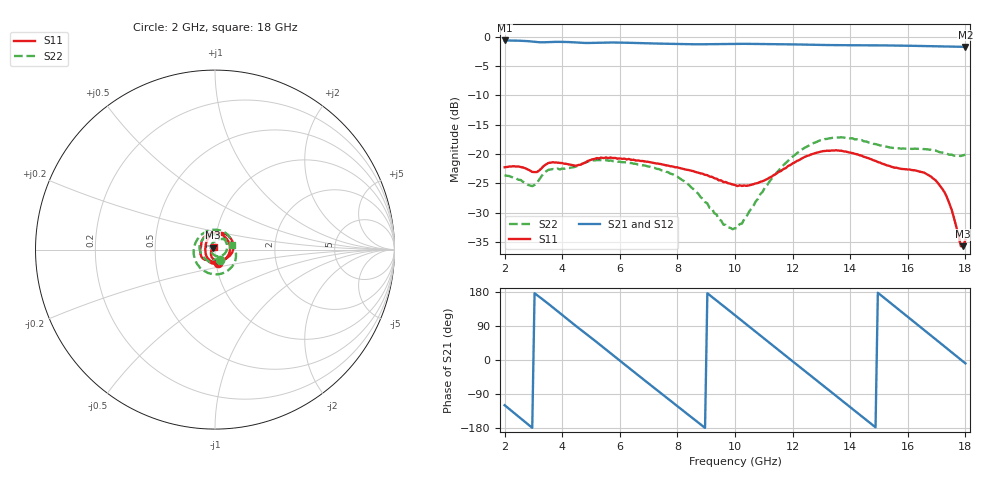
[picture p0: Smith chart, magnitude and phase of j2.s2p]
!Keysight Technologies,P5004A,MY58100454,A.15.10.06
!Date: Monday, July 18, 2022 10:32:16
!Correction: S11(C  2-Port  )
!S21(C  2-Port  )
!S12(C  2-Port  )
!S22(C  2-Port  )
!S2P File: Measurements: S11, S21, S12, S22:
# Hz S  dB  R 50
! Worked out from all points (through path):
!   201 points, 2 GHz to 18 GHz, reference 50 ohm
!   highest |S21| = -0.66 dB at 2 GHz (marker M1); lowest = -1.8 dB at 18 GHz (marker M2)
!   group delay of S21, straight-line fit = 168 ps
!   lowest |S11| = -35.7 dB at 17.92 GHz (marker M3), VSWR 1.03, Z = 48.7 + j1.01 ohm
!   |S11| at or under -10 dB: start of sweep to end of sweep
!   |S22| runs from -32.8 to -17.2 dB; largest |S21 - S12| = 0.00052
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2e9  -22.24 -76.1  -0.66 -119.2  -0.66 -119.2  -23.60 -63.9
2.64e9  -22.28 -111.1  -0.73 -159.1  -0.73 -159.1  -24.73 -89.6
3.2e9  -22.79 -128.3  -0.96 166.9  -0.96 166.9  -24.35 -94.0
4e9  -21.54 -171.1  -0.90 118.9  -0.90 118.9  -22.45 -137.3
4.72e9  -21.59 157.1  -1.08 75.3  -1.08 75.3  -21.58 -173.3
6e9  -20.73 79.7  -1.02 -1.5  -1.02 -1.6  -21.29 109.0
6.56e9  -21.11 45.0  -1.09 -35.6  -1.09 -35.6  -21.66 77.0
7.36e9  -21.64 -5.7  -1.19 -83.6  -1.19 -83.6  -22.56 31.8
8e9  -22.27 -47.1  -1.26 -122.0  -1.26 -122.0  -23.85 -6.1
8.8e9  -23.29 -100.2  -1.31 -169.6  -1.31 -169.6  -27.28 -57.8
1e10  -25.25 -169.0  -1.24 118.2  -1.24 118.2  -32.62 -173.7
1.072e10  -25.00 160.4  -1.25 74.4  -1.25 74.4  -28.06 108.8
1.152e10  -23.02 126.0  -1.29 25.8  -1.29 25.8  -22.78 54.0
1.208e10  -21.41 100.5  -1.33 -8.2  -1.33 -8.2  -20.15 19.6
1.272e10  -19.94 67.8  -1.40 -47.0  -1.39 -47.0  -18.15 -19.4
1.384e10  -19.57 12.9  -1.47 -114.5  -1.47 -114.5  -17.25 -90.3
1.464e10  -20.71 -18.0  -1.48 -163.1  -1.48 -163.1  -18.02 -147.3
1.536e10  -22.01 -39.0  -1.51 153.0  -1.51 153.0  -18.87 155.1
1.656e10  -23.14 -72.1  -1.61 79.5  -1.61 79.5  -19.14 62.5
1.728e10  -26.54 -111.9  -1.68 35.4  -1.68 35.4  -19.82 27.3
1.792e10  -35.67 141.0  -1.75 -4.0  -1.75 -4.0  -20.22 15.3
1.8e10  -34.61 112.0  -1.75 -8.9  -1.75 -8.9  -20.09 15.1
